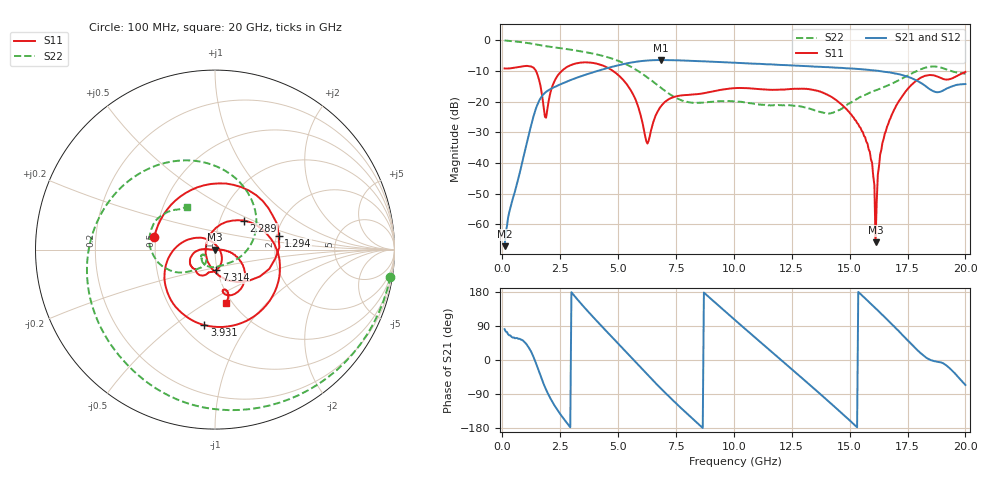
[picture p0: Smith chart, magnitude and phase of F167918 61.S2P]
!  2-Port S-parameters saved by WinCal
! VAR MeasName=S-Parameters (CALIBRATED_DATA) read from VNA (N5242A)
! VAR MeasDate=2016-11-22 10:27:51
! VAR NAME=F167918 61
! VAR FILENAME=F167918 61.S2P
! VAR DATE=2016-11-22 10:27:51
! VAR PHYS_PORTS=1,2
# Hz S DB R 50
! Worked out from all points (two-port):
!   401 points, 100 MHz to 20 GHz, reference 50 ohm
!   highest |S21| = -6.48 dB at 6.866 GHz (marker M1); lowest = -67.2 dB at 100 MHz (marker M2)
!   |S21| within 3 dB of the highest: 4.361 GHz to 15.46 GHz (11.1 GHz wide, 112 % of centre)
!   lowest |S11| = -65.8 dB at 16.12 GHz (marker M3), VSWR 1.00, Z = 50 - j0.0409 ohm
!   |S11| at or under -10 dB: 1.451 GHz to 2.578 GHz (1.126 GHz wide, 55.9 % of centre); 4.773 GHz to end of sweep
!   |S22| runs from -24.0 to -0.1 dB; largest |S21 - S12| = 0.0043
!   S11 on the Smith chart (normalised r, x): 100 MHz: 0.49, +0.08; 1.294 GHz: 2.06, +0.37; 2.289 GHz: 1.30, +0.44; 3.931 GHz: 0.63, -0.65; 7.314 GHz: 0.99, -0.23; 20 GHz: 0.93, -0.61
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1e8  -9.22 168.4  -67.17 81.5  -66.03 80.0  -0.10 -8.8
7.965e8  -8.65 87.2  -41.86 54.2  -41.92 54.5  -0.63 -63.5
1.294e9  -8.80 12.3  -26.39 15.6  -26.43 16.0  -1.16 -97.8
1.891e9  -25.28 157.0  -16.85 -78.1  -16.84 -77.9  -1.98 -132.0
2.289e9  -12.80 45.0  -15.19 -123.1  -15.20 -123.0  -2.39 -151.6
3.43325e9  -7.28 -62.7  -11.67 146.4  -11.63 146.8  -3.69 157.6
3.93075e9  -7.43 -98.0  -10.46 112.8  -10.39 113.0  -4.41 136.5
5.42325e9  -14.89 165.7  -7.50 16.2  -7.48 15.9  -8.14 67.5
6.269e9  -33.71 38.3  -6.64 -38.6  -6.65 -38.8  -12.17 23.7
6.7665e9  -22.53 -60.5  -6.48 -70.1  -6.50 -70.1  -15.05 -1.7
6.866e9  -21.44 -66.6  -6.48 -76.1  -6.50 -76.2  -15.61 -6.8
7.31375e9  -18.81 -86.5  -6.53 -103.1  -6.52 -103.1  -18.00 -28.5
8.60725e9  -17.44 -106.6  -6.87 -176.6  -6.85 -176.6  -20.37 -83.1
1.005e10  -15.63 -120.5  -7.35 105.3  -7.34 105.3  -19.98 -129.5
1.179125e10  -16.19 -134.0  -7.98 13.3  -7.96 13.2  -21.22 -149.1
1.338325e10  -16.18 -153.7  -8.55 -71.2  -8.52 -71.2  -22.61 -158.1
1.547275e10  -28.59 176.5  -9.49 174.0  -9.50 173.8  -18.50 -126.8
1.587075e10  -36.38 -178.8  -9.73 150.9  -9.76 151.0  -17.14 -131.2
1.61195e10  -65.85 -126.6  -9.90 136.8  -9.97 136.6  -16.37 -133.2
1.67165e10  -26.17 -2.7  -10.49 101.1  -10.56 101.3  -14.58 -139.5
1.801e10  -12.53 -45.8  -13.66 21.5  -13.56 21.8  -9.69 -168.4
2e10  -10.35 -78.5  -14.31 -66.1  -14.18 -66.0  -10.94 123.0
